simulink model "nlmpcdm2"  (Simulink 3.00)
settings: Solver=ode45  SolverMode=SingleTasking  StartTime=0.0  StopTime=30  FixedStep=[]  MaxStep=2  RelTol=1e-3  AbsTol=1e-3
PreLoadFcn:
  | demo2dat
libraries: nlmpclib x1

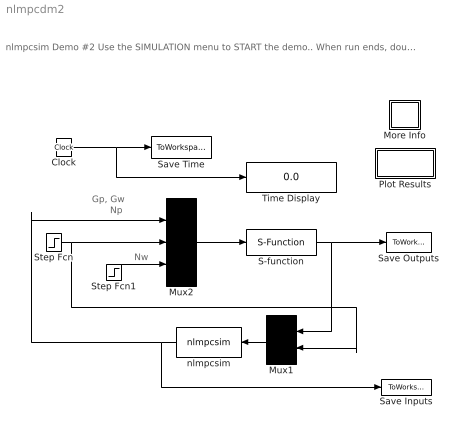
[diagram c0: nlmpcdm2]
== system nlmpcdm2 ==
  note: Gp, Gw
  note: Np
  note: Nw
  note: nlmpcsim Demo #2 Use the SIMULATION menu to START the demo.. When run ends, double click on PLOT RESULTS. (Double click on the "?" for more info)
  Clock : Clock
  More Info : Subsystem
  Mux1 : Mux  Orientation=left  Inputs=[3 1]
  Mux2 : Mux  Inputs=[2 1 1]
  Plot Results : Subsystem
  S-function : S-Function  FunctionName=papmach  PortCounts=[]  SFunctionModules=''
  Save Inputs : ToWorkspace  VariableName=u  SampleTime=0
  Save Outputs : ToWorkspace  VariableName=y  SampleTime=0
  Save Time : ToWorkspace  VariableName=t  SampleTime=0
  Step Fcn : Step  Time=0  Before=0  After=1  SampleTime=0
  Step Fcn1 : Step  Time=0  Before=0  After=0  SampleTime=0
  Time Display : Display
  nlmpcsim : nlmpclib/nlmpcsim  Orientation=left
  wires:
  Clock/1 -> Save Time/1, Time Display/1
  Mux2/1 -> S-function/1
  Step Fcn1/1 -> Mux2/3
  Step Fcn/1 -> Mux1/2, Mux2/2
  S-function/1 -> Save Outputs/1, Mux1/1
  Mux1/1 -> nlmpcsim/1
  nlmpcsim/1 -> Mux2/1, Save Inputs/1

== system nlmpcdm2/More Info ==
  note: This demonstration shows how NLMPCSIM works. The plant is the paper machine headbox discussed in Section 3.4 of the MPC Tools manual. See NLMPCSIM in Command Reference for details
  note: Use the Simulation menu to Start the demo. At the end of the simulation, double-click on "Plot Results" to have inputs and outputs displayed in a figure window using the MPC Tools PLOTEACH command.

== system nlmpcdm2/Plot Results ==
